| IBIS file stm32u5f9_5g9_lqfp144_dsi_smps.ibs
[IBIS ver] 4.2
[File name] stm32u5f9_5g9_lqfp144_dsi_smps.ibs
[File Rev] 1.0
[Date]  29-10-2024
[Source] Data Created at STMicroelectronics
[Notes]  File originated from ELDO simulations.
[Disclaimer]  This information is for modeling purpose only and is
   not guaranteed. The information is subject to change without
   notice.
[Copyright] Copyright 2024 STMicroelectronics Inc.
|   Component stm32u5f9_5g9_lqfp144_dsi_smps
[Component] stm32u5f9_5g9_lqfp144_dsi_smps
[Manufacturer] STMicroelectronics
[Package]
| variable   typ   min   max
R_pkg  0  NA  NA
L_pkg  0  NA  NA
C_pkg  0  NA  NA
[Pin]   signal_name   model_name
1 PE2 io8_100m_hslv_ft
2 PE3 io8_100m_hslv_tamp_ft
3 PE4 io8_100m_hslv_tamp_ft
4 PE5 io8_100m_hslv_tamp_ft
5 PE6 io8_100m_hslv_tamp_ft
6 VBAT power
7 PC13 io8_100m_ft_v33
8 PC14-OSC32_IN  io8_100m_ft
9 PC15-OSC32_OUT io8_100m_ft
10 PF0 io8_100m_hslv_ft
11 PF1 io8_100m_hslv_ft
12 PF2 io8_100m_hslv_ft
13 VDDDSI nc
14 VDD11DSI nc
15 DSI_D0P nc
16 DSI_D0N nc
17 VSSDSI nc
18 DSI_CKP nc
19 DSI_CKN nc
20 VDD11DSI nc
21 DSI_D1P nc
22 DSI_D1N nc
23 VSSDSI nc
24 VSS gnd
25 VDD power
26 PH0-OSC_IN io8_100m_ft
27 PH1-OSC_OUT io8_100m_ft
28 NRST nc
29 PC0 io8_100m_hslv_ft
30 PC1 io8_166m_hslv_i2c_ft
31 PC2 io8_100m_hslv_ft
32 PC3 io8_100m_hslv_ft
33 VSSA nc
34 VREFP nc
35 VDDA nc
36 PA0 io8_100m_hslv_tamp_ft
37 PA1 io8_100m_hslv_tamp_ft
38 PA2 io8_100m_hslv_ft
39 PA3 io8_166m_hslv_ft
40 VSS gnd
41 VDD power
42 PA4 io8_100m_hslv_ft
43 PA5 io8_100m_ft
44 PA6 io8_100m_hslv_ft
45 PA7 io8_100m_hslv_ft
46 PB0 io8_100m_hslv_ft
47 PB1 io8_100m_hslv_ft
48 PB2 io8_100m_hslv_tamp_ft
49 PG0 io8_100m_hslv_ft
50 PG1 io8_100m_hslv_ft
51 PE7 io8_100m_hslv_ft
52 PE8 io8_100m_hslv_ft
53 PE9 io8_166m_hslv_ft
54 VSS gnd
55 VDD power
56 PE10 io8_166m_hslv_ft
57 PE11 io8_100m_hslv_ft
58 PE12 io8_100m_hslv_ft
59 PE13 io8_100m_hslv_ft
60 PE14 io8_100m_hslv_ft
61 PE15 io8_100m_hslv_ft
62 PB10 io8_166m_hslv_i2c_ft
63 PB11 io8_100m_hslv_ft
64 VLXSMPS nc
65 VDDSMPS nc
66 VSSSMPS nc
67 VDD11 nc
68 VSS gnd
69 VDD power
70 PB13 io8_100m_i2c_ft
71 PB14 io8_100m_hslv_ft
72 PB15 nc
73 PD8 io8_100m_hslv_ft
74 PD9 io8_100m_hslv_ft
75 PD10 io8_100m_hslv_ft
76 PD11 io8_100m_hslv_ft
77 PD12 io8_100m_hslv_ft
78 PD13 io8_100m_hslv_ft
79 PD14 io8_100m_hslv_ft
80 PD15 io8_100m_hslv_ft
81 PH9 io8_spi_ft
82 VSS gnd
83 VDD power
84 PH10 io8_spi_ft
85 PH11 io8_spi_ft
86 PH12 io8_spi_ft
87 PH13 io8_spi_ft
88 VSS gnd
89 VDD power
90 PH14 io8_spi_ft
91 PH15 io8_spi_ft
92 PI0 io8_spi_ft
93 PI1 io8_spi_ft
94 VSS gnd
95 VDD power
96 PI2 io8_spi_ft
97 PI3 io8_spi_ft
98 PC6 io8_100m_hslv_ft
99 PC7 io8_100m_hslv_ft
100 PC8 io8_100m_hslv_ft
101 PC9 io8_100m_hslv_ft
102 PA8 io8_166m_hslv_ft
103 PA9 io8_100m_usb_vbus_ft
104 PA10 io8_100m_usb_id
105 PA11 io8_100m_ft
106 PA12 io8_100m_ft
107 PA13 io8_100m_ft
108 VDDUSB power
109 VDD power
110 VSS gnd
111 PA14 io8_100m_ft
112 PA15 nc
113 PC10 io8_100m_hslv_ft
114 PC11 io8_100m_hslv_ft
115 PC12 io8_166m_hslv_ft
116 PD0 io8_100m_hslv_ft
117 PD1 io8_100m_hslv_ft
118 PD2 io8_100m_hslv_ft
119 PD3 io8_166m_hslv_ft
120 PD4 io8_100m_hslv_ft
121 PD5 io8_100m_hslv_ft
122 VDD power
123 PD6 io8_166m_hslv_ft
124 PD7 io8_100m_hslv_ft
125 PG9 io8_100m_hslv_ft
126 PG10 io8_100m_hslv_ft
127 PG12 io8_100m_hslv_ft
128 PG13 io8_100m_hslv_ft
129 PG14 io8_100m_hslv_ft
130 VSS gnd
131 VDDIO2 power
132 PG15 io8_100m_hslv_ft
133 PB3 io8_100m_hslv_ft
134 PB4 io8_100m_hslv_ft
135 PB5 io8_166m_hslv_ft
136 PB6 io8_100m_i2c_ft
137 PB7 io8_166m_hslv_i2c_ft
138 PH3-BOOT0 io8_100m_ft
139 PB8 io8_100m_hslv_ft
140 PB9 io8_100m_hslv_ft
141 PE0 io8_100m_hslv_ft
142 VDD11 nc
143 VSS gnd
144 VDD power
[Package Model]   476-lqfp-20x20-144-smps-dsi-220916
[Pin Mapping]   pulldown_ref   pullup_ref   | Comment
19  nc  nc
18  nc  nc
16  nc  nc
15  nc  nc
22  nc  nc
21  nc  nc
28  nc  nc
36  gndio  vddiom
37  gndio  vddiom
104  gndio  vddiom  | Depending on IO usage
| 104  gndio  vddusb  | Depending on IO usage
105  gndio  vddiom  | Depending on IO usage
| 105  gndio  vddusb  | Depending on IO usage
106  gndio  vddiom  | Depending on IO usage
| 106  gndio  vddusb  | Depending on IO usage
107  gndio  vddiom  | Depending on IO usage
| 107  gndio  vddusb  | Depending on IO usage
111  gndio  vddiom
112  nc  nc
38  gndio  vddiom
39  gndio  vddiom
42  gndio  vddiom
43  gndio  vddiom
44  gndio  vddiom
45  gndio  vddiom
102  gndio  vddiom
103  gndio  vddiom  | Depending on IO usage
| 103  gndio  vddusb  | Depending on IO usage
46  gndio  vddiom
47  gndio  vddiom
62  gndio  vddiom
63  gndio  vddiom
70  gndio  vddiom
71  gndio  vddiom
72  nc  nc
48  gndio  vddiom
133  gndio  vddiom
134  gndio  vddiom
135  gndio  vddiom
136  gndio  vddiom
137  gndio  vddiom
139  gndio  vddiom
140  gndio  vddiom
29  gndio  vddiom
30  gndio  vddiom
113  gndio  vddiom
114  gndio  vddiom
115  gndio  vddiom
7  gndio  vddiom  | Depending on IO usage
| 7  gndio  vsw  | Depending on IO usage
8  gndio  vddiom  | Depending on IO usage
| 8  gndio  vsw  | Depending on IO usage
9  gndio  vddiom  | Depending on IO usage
| 9  gndio  vsw  | Depending on IO usage
31  gndio  vddiom
32  gndio  vddiom
98  gndio  vddiom
99  gndio  vddiom
100  gndio  vddiom
101  gndio  vddiom
116  gndio  vddiom
117  gndio  vddiom
75  gndio  vddiom
76  gndio  vddiom
77  gndio  vddiom
78  gndio  vddiom
79  gndio  vddiom
80  gndio  vddiom
118  gndio  vddiom
119  gndio  vddiom
120  gndio  vddiom
121  gndio  vddiom
123  gndio  vddiom
124  gndio  vddiom
73  gndio  vddiom
74  gndio  vddiom
141  gndio  vddiom
56  gndio  vddiom
57  gndio  vddiom
58  gndio  vddiom
59  gndio  vddiom
60  gndio  vddiom
61  gndio  vddiom
1  gndio  vddiom
2  gndio  vddiom
3  gndio  vddiom
4  gndio  vddiom
5  gndio  vddiom
51  gndio  vddiom
52  gndio  vddiom
53  gndio  vddiom
10  gndio  vddiom
11  gndio  vddiom
12  gndio  vddiom
49  gndio  vddiom
50  gndio  vddiom
126  gndio  vddiom  | Depending on IO usage
| 126  gndio  vddio2  | Depending on IO usage
127  gndio  vddiom  | Depending on IO usage
| 127  gndio  vddio2  | Depending on IO usage
128  gndio  vddiom  | Depending on IO usage
| 128  gndio  vddio2  | Depending on IO usage
129  gndio  vddiom  | Depending on IO usage
| 129  gndio  vddio2  | Depending on IO usage
132  gndio  vddiom  | Depending on IO usage
| 132  gndio  vddio2  | Depending on IO usage
125  gndio  vddiom  | Depending on IO usage
| 125  gndio  vddio2  | Depending on IO usage
26  gndio  vddiom
27  gndio  vddiom
84  gndio  vddiom
85  gndio  vddiom  | Depending on IO usage
| 85  gndio  vddhspi  | Depending on IO usage
86  gndio  vddiom  | Depending on IO usage
| 86  gndio  vddhspi  | Depending on IO usage
87  gndio  vddiom  | Depending on IO usage
| 87  gndio  vddhspi  | Depending on IO usage
90  gndio  vddiom  | Depending on IO usage
| 90  gndio  vddhspi  | Depending on IO usage
91  gndio  vddiom  | Depending on IO usage
| 91  gndio  vddhspi  | Depending on IO usage
138  gndio  vddiom
81  gndio  vddiom  | Depending on IO usage
| 81  gndio  vddhspi  | Depending on IO usage
92  gndio  vddiom  | Depending on IO usage
| 92  gndio  vddhspi  | Depending on IO usage
93  gndio  vddiom  | Depending on IO usage
| 93  gndio  vddhspi  | Depending on IO usage
96  gndio  vddiom  | Depending on IO usage
| 96  gndio  vddhspi  | Depending on IO usage
97  gndio  vddiom  | Depending on IO usage
| 97  gndio  vddhspi  | Depending on IO usage
67  nc  nc
142  nc  nc
6  nc  vsw
83  nc  vddhspi
89  nc  vddhspi
95  nc  vddhspi
13  nc  nc
109  nc  vddiom
14  nc  nc
20  nc  nc
122  nc  vddiom
144  nc  vddiom
25  nc  vddiom
108  nc  vddusb
41  nc  vddiom
55  nc  vddiom
69  nc  vddiom
35  nc  nc
131  nc  vddio2
65  nc  nc
64  nc  nc
34  nc  nc
24  gndio  nc
40  gndio  nc
54  gndio  nc
68  gndio  nc
110  gndio  nc
143  gndio  nc
17  nc  nc
23  nc  nc
130  gndio  nc
82  gndio  nc
88  gndio  nc
94  gndio  nc
33  nc  nc
66  nc  nc
[Model Selector] io8_100m_ft
io8_100m_ft_hs_1v2  "IO8_FT 100MHz high speed @ 1.2V"
io8_100m_ft_fs_1v2  "IO8_FT 100MHz fast speed @ 1.2V"
io8_100m_ft_fs_pd_1v2  "IO8_FT 100MHz fast speed @ 1.2V pulldown"
io8_100m_ft_ms_1v2  "IO8_FT 100MHz med speed @ 1.2V"
io8_100m_ft_ms_pd_1v2  "IO8_FT 100MHz med speed @ 1.2V pulldown"
io8_100m_ft_ls_1v2  "IO8_FT 100MHz low speed @ 1.2V"
io8_100m_ft_ls_pd_1v2  "IO8_FT 100MHz low speed @ 1.2V pulldown"
io8_100m_ft_hs_1v8  "IO8_FT 100MHz high speed @ 1.8V"
io8_100m_ft_hs_pd_1v8  "IO8_FT 100MHz high speed @ 1.8V pulldown"
io8_100m_ft_fs_1v8  "IO8_FT 100MHz fast speed @ 1.8V"
io8_100m_ft_fs_pd_1v8  "IO8_FT 100MHz fast speed @ 1.8V pulldown"
io8_100m_ft_ms_1v8  "IO8_FT 100MHz med speed @ 1.8V"
io8_100m_ft_ms_pd_1v8  "IO8_FT 100MHz med speed @ 1.8V pulldown"
io8_100m_ft_ls_1v8  "IO8_FT 100MHz low speed @ 1.8V"
io8_100m_ft_ls_pd_1v8  "IO8_FT 100MHz low speed @ 1.8V pulldown"
io8_100m_ft_hs_3v3  "IO8_FT 100MHz high speed @ 3.3V"
io8_100m_ft_hs_pd_3v3  "IO8_FT 100MHz high speed @ 3.3V pulldown"
io8_100m_ft_fs_3v3  "IO8_FT 100MHz fast speed @ 3.3V"
io8_100m_ft_fs_pd_3v3  "IO8_FT 100MHz fast speed @ 3.3V pulldown"
io8_100m_ft_ms_3v3  "IO8_FT 100MHz med speed @ 3.3V"
io8_100m_ft_ms_pd_3v3  "IO8_FT 100MHz med speed @ 3.3V pulldown"
io8_100m_ft_ls_3v3  "IO8_FT 100MHz low speed @ 3.3V"
io8_100m_ft_ls_pd_3v3  "IO8_FT 100MHz low speed @ 3.3V pulldown"
[Model Selector] io8_100m_hslv_ft
io8_100m_ft_hs_1v2  "IO8_FT 100MHz high speed @ 1.2V"
io8_100m_ft_hs_pu_1v2  "IO8_FT 100MHz high speed @ 1.2V pullup"
io8_100m_ft_hs_pd_1v2  "IO8_FT 100MHz high speed @ 1.2V pulldown"
io8_100m_ft_fs_1v2  "IO8_FT 100MHz fast speed @ 1.2V"
io8_100m_ft_fs_pu_1v2  "IO8_FT 100MHz fast speed @ 1.2V pullup"
io8_100m_ft_fs_pd_1v2  "IO8_FT 100MHz fast speed @ 1.2V pulldown"
io8_100m_ft_ms_1v2  "IO8_FT 100MHz med speed @ 1.2V"
io8_100m_ft_ms_pu_1v2  "IO8_FT 100MHz med speed @ 1.2V pullup"
io8_100m_ft_ms_pd_1v2  "IO8_FT 100MHz med speed @ 1.2V pulldown"
io8_100m_ft_ls_1v2  "IO8_FT 100MHz low speed @ 1.2V"
io8_100m_ft_ls_pu_1v2  "IO8_FT 100MHz low speed @ 1.2V pullup"
io8_100m_ft_ls_pd_1v2  "IO8_FT 100MHz low speed @ 1.2V pulldown"
io8_100m_ft_hs_1v8  "IO8_FT 100MHz high speed @ 1.8V"
io8_100m_ft_hs_pu_1v8  "IO8_FT 100MHz high speed @ 1.8V pullup"
io8_100m_ft_hs_pd_1v8  "IO8_FT 100MHz high speed @ 1.8V pulldown"
io8_100m_ft_fs_1v8  "IO8_FT 100MHz fast speed @ 1.8V"
io8_100m_ft_fs_pu_1v8  "IO8_FT 100MHz fast speed @ 1.8V pullup"
io8_100m_ft_fs_pd_1v8  "IO8_FT 100MHz fast speed @ 1.8V pulldown"
io8_100m_ft_ms_1v8  "IO8_FT 100MHz med speed @ 1.8V"
io8_100m_ft_ms_pu_1v8  "IO8_FT 100MHz med speed @ 1.8V pullup"
io8_100m_ft_ms_pd_1v8  "IO8_FT 100MHz med speed @ 1.8V pulldown"
io8_100m_ft_ls_1v8  "IO8_FT 100MHz low speed @ 1.8V"
io8_100m_ft_ls_pu_1v8  "IO8_FT 100MHz low speed @ 1.8V pullup"
io8_100m_ft_ls_pd_1v8  "IO8_FT 100MHz low speed @ 1.8V pulldown"
io8_100m_ft_hs_3v3  "IO8_FT 100MHz high speed @ 3.3V"
io8_100m_ft_hs_pu_3v3  "IO8_FT 100MHz high speed @ 3.3V pullup"
io8_100m_ft_hs_pd_3v3  "IO8_FT 100MHz high speed @ 3.3V pulldown"
io8_100m_ft_fs_3v3  "IO8_FT 100MHz fast speed @ 3.3V"
io8_100m_ft_fs_pu_3v3  "IO8_FT 100MHz fast speed @ 3.3V pullup"
io8_100m_ft_fs_pd_3v3  "IO8_FT 100MHz fast speed @ 3.3V pulldown"
io8_100m_ft_ms_3v3  "IO8_FT 100MHz med speed @ 3.3V"
io8_100m_ft_ms_pu_3v3  "IO8_FT 100MHz med speed @ 3.3V pullup"
io8_100m_ft_ms_pd_3v3  "IO8_FT 100MHz med speed @ 3.3V pulldown"
io8_100m_ft_ls_3v3  "IO8_FT 100MHz low speed @ 3.3V"
io8_100m_ft_ls_pu_3v3  "IO8_FT 100MHz low speed @ 3.3V pullup"
io8_100m_ft_ls_pd_3v3  "IO8_FT 100MHz low speed @ 3.3V pulldown"
io8_100m_hslv_ft_hs_1v2  "IO8_FT 100MHz HSLV high speed @ 1.2V"
io8_100m_hslv_ft_hs_pu_1v2  "IO8_FT 100MHz HSLV high speed @ 1.2V pullup"
io8_100m_hslv_ft_hs_pd_1v2  "IO8_FT 100MHz HSLV high speed @ 1.2V pulldown"
io8_100m_hslv_ft_fs_1v2  "IO8_FT 100MHz HSLV fast speed @ 1.2V"
io8_100m_hslv_ft_fs_pu_1v2  "IO8_FT 100MHz HSLV fast speed @ 1.2V pullup"
io8_100m_hslv_ft_fs_pd_1v2  "IO8_FT 100MHz HSLV fast speed @ 1.2V pulldown"
io8_100m_hslv_ft_ms_1v2  "IO8_FT 100MHz HSLV med speed @ 1.2V"
io8_100m_hslv_ft_ms_pu_1v2  "IO8_FT 100MHz HSLV med speed @ 1.2V pullup"
io8_100m_hslv_ft_ms_pd_1v2  "IO8_FT 100MHz HSLV med speed @ 1.2V pulldown"
io8_100m_hslv_ft_ls_1v2  "IO8_FT 100MHz HSLV low speed @ 1.2V"
io8_100m_hslv_ft_ls_pu_1v2  "IO8_FT 100MHz HSLV low speed @ 1.2V pullup"
io8_100m_hslv_ft_ls_pd_1v2  "IO8_FT 100MHz HSLV low speed @ 1.2V pulldown"
io8_100m_hslv_ft_hs_1v8  "IO8_FT 100MHz HSLV high speed @ 1.8V"
io8_100m_hslv_ft_hs_pu_1v8  "IO8_FT 100MHz HSLV high speed @ 1.8V pullup"
io8_100m_hslv_ft_hs_pd_1v8  "IO8_FT 100MHz HSLV high speed @ 1.8V pulldown"
io8_100m_hslv_ft_fs_1v8  "IO8_FT 100MHz HSLV fast speed @ 1.8V"
io8_100m_hslv_ft_fs_pu_1v8  "IO8_FT 100MHz HSLV fast speed @ 1.8V pullup"
io8_100m_hslv_ft_fs_pd_1v8  "IO8_FT 100MHz HSLV fast speed @ 1.8V pulldown"
io8_100m_hslv_ft_ms_1v8  "IO8_FT 100MHz HSLV med speed @ 1.8V"
io8_100m_hslv_ft_ms_pu_1v8  "IO8_FT 100MHz HSLV med speed @ 1.8V pullup"
io8_100m_hslv_ft_ms_pd_1v8  "IO8_FT 100MHz HSLV med speed @ 1.8V pulldown"
io8_100m_hslv_ft_ls_1v8  "IO8_FT 100MHz HSLV low speed @ 1.8V"
io8_100m_hslv_ft_ls_pu_1v8  "IO8_FT 100MHz HSLV low speed @ 1.8V pullup"
io8_100m_hslv_ft_ls_pd_1v8  "IO8_FT 100MHz HSLV low speed @ 1.8V pulldown"
io8_100m_hslv_ft_hs_2v5  "IO8_FT 100MHz HSLV high speed @ 2.5V"
io8_100m_hslv_ft_hs_pu_2v5  "IO8_FT 100MHz HSLV high speed @ 2.5V pullup"
io8_100m_hslv_ft_hs_pd_2v5  "IO8_FT 100MHz HSLV high speed @ 2.5V pulldown"
io8_100m_hslv_ft_fs_2v5  "IO8_FT 100MHz HSLV fast speed @ 2.5V"
io8_100m_hslv_ft_fs_pu_2v5  "IO8_FT 100MHz HSLV fast speed @ 2.5V pullup"
io8_100m_hslv_ft_fs_pd_2v5  "IO8_FT 100MHz HSLV fast speed @ 2.5V pulldown"
io8_100m_hslv_ft_ms_2v5  "IO8_FT 100MHz HSLV med speed @ 2.5V"
io8_100m_hslv_ft_ms_pu_2v5  "IO8_FT 100MHz HSLV med speed @ 2.5V pullup"
io8_100m_hslv_ft_ms_pd_2v5  "IO8_FT 100MHz HSLV med speed @ 2.5V pulldown"
io8_100m_hslv_ft_ls_2v5  "IO8_FT 100MHz HSLV low speed @ 2.5V"
io8_100m_hslv_ft_ls_pu_2v5  "IO8_FT 100MHz HSLV low speed @ 2.5V pullup"
io8_100m_hslv_ft_ls_pd_2v5  "IO8_FT 100MHz HSLV low speed @ 2.5V pulldown"
[Model Selector] io8_100m_hslv_tamp_ft
io8_100m_ft_hs_1v2  "IO8_FT 100MHz high speed @ 1.2V"
io8_100m_ft_hs_pu_1v2  "IO8_FT 100MHz high speed @ 1.2V pullup"
io8_100m_ft_hs_pd_1v2  "IO8_FT 100MHz high speed @ 1.2V pulldown"
io8_100m_ft_fs_1v2  "IO8_FT 100MHz fast speed @ 1.2V"
io8_100m_ft_fs_pu_1v2  "IO8_FT 100MHz fast speed @ 1.2V pullup"
io8_100m_ft_fs_pd_1v2  "IO8_FT 100MHz fast speed @ 1.2V pulldown"
io8_100m_ft_ms_1v2  "IO8_FT 100MHz med speed @ 1.2V"
io8_100m_ft_ms_pu_1v2  "IO8_FT 100MHz med speed @ 1.2V pullup"
io8_100m_ft_ms_pd_1v2  "IO8_FT 100MHz med speed @ 1.2V pulldown"
io8_100m_ft_ls_1v2  "IO8_FT 100MHz low speed @ 1.2V"
io8_100m_ft_ls_pu_1v2  "IO8_FT 100MHz low speed @ 1.2V pullup"
io8_100m_ft_ls_pd_1v2  "IO8_FT 100MHz low speed @ 1.2V pulldown"
io8_100m_ft_hs_1v8  "IO8_FT 100MHz high speed @ 1.8V"
io8_100m_ft_hs_pu_1v8  "IO8_FT 100MHz high speed @ 1.8V pullup"
io8_100m_ft_hs_pd_1v8  "IO8_FT 100MHz high speed @ 1.8V pulldown"
io8_100m_ft_fs_1v8  "IO8_FT 100MHz fast speed @ 1.8V"
io8_100m_ft_fs_pu_1v8  "IO8_FT 100MHz fast speed @ 1.8V pullup"
io8_100m_ft_fs_pd_1v8  "IO8_FT 100MHz fast speed @ 1.8V pulldown"
io8_100m_ft_ms_1v8  "IO8_FT 100MHz med speed @ 1.8V"
io8_100m_ft_ms_pu_1v8  "IO8_FT 100MHz med speed @ 1.8V pullup"
io8_100m_ft_ms_pd_1v8  "IO8_FT 100MHz med speed @ 1.8V pulldown"
io8_100m_ft_ls_1v8  "IO8_FT 100MHz low speed @ 1.8V"
io8_100m_ft_ls_pu_1v8  "IO8_FT 100MHz low speed @ 1.8V pullup"
io8_100m_ft_ls_pd_1v8  "IO8_FT 100MHz low speed @ 1.8V pulldown"
io8_100m_ft_hs_3v3  "IO8_FT 100MHz high speed @ 3.3V"
io8_100m_ft_hs_pu_3v3  "IO8_FT 100MHz high speed @ 3.3V pullup"
io8_100m_ft_hs_pd_3v3  "IO8_FT 100MHz high speed @ 3.3V pulldown"
io8_100m_ft_fs_3v3  "IO8_FT 100MHz fast speed @ 3.3V"
io8_100m_ft_fs_pu_3v3  "IO8_FT 100MHz fast speed @ 3.3V pullup"
io8_100m_ft_fs_pd_3v3  "IO8_FT 100MHz fast speed @ 3.3V pulldown"
io8_100m_ft_ms_3v3  "IO8_FT 100MHz med speed @ 3.3V"
io8_100m_ft_ms_pu_3v3  "IO8_FT 100MHz med speed @ 3.3V pullup"
io8_100m_ft_ms_pd_3v3  "IO8_FT 100MHz med speed @ 3.3V pulldown"
io8_100m_ft_ls_3v3  "IO8_FT 100MHz low speed @ 3.3V"
io8_100m_ft_ls_pu_3v3  "IO8_FT 100MHz low speed @ 3.3V pullup"
io8_100m_ft_ls_pd_3v3  "IO8_FT 100MHz low speed @ 3.3V pulldown"
io8_100m_hslv_ft_hs_1v2  "IO8_FT 100MHz HSLV high speed @ 1.2V"
io8_100m_hslv_ft_hs_pu_1v2  "IO8_FT 100MHz HSLV high speed @ 1.2V pullup"
io8_100m_hslv_ft_hs_pd_1v2  "IO8_FT 100MHz HSLV high speed @ 1.2V pulldown"
io8_100m_hslv_ft_fs_1v2  "IO8_FT 100MHz HSLV fast speed @ 1.2V"
io8_100m_hslv_ft_fs_pu_1v2  "IO8_FT 100MHz HSLV fast speed @ 1.2V pullup"
io8_100m_hslv_ft_fs_pd_1v2  "IO8_FT 100MHz HSLV fast speed @ 1.2V pulldown"
io8_100m_hslv_ft_ms_1v2  "IO8_FT 100MHz HSLV med speed @ 1.2V"
io8_100m_hslv_ft_ms_pu_1v2  "IO8_FT 100MHz HSLV med speed @ 1.2V pullup"
io8_100m_hslv_ft_ms_pd_1v2  "IO8_FT 100MHz HSLV med speed @ 1.2V pulldown"
io8_100m_hslv_ft_ls_1v2  "IO8_FT 100MHz HSLV low speed @ 1.2V"
io8_100m_hslv_ft_ls_pu_1v2  "IO8_FT 100MHz HSLV low speed @ 1.2V pullup"
io8_100m_hslv_ft_ls_pd_1v2  "IO8_FT 100MHz HSLV low speed @ 1.2V pulldown"
io8_100m_hslv_ft_hs_1v8  "IO8_FT 100MHz HSLV high speed @ 1.8V"
io8_100m_hslv_ft_hs_pu_1v8  "IO8_FT 100MHz HSLV high speed @ 1.8V pullup"
io8_100m_hslv_ft_hs_pd_1v8  "IO8_FT 100MHz HSLV high speed @ 1.8V pulldown"
io8_100m_hslv_ft_fs_1v8  "IO8_FT 100MHz HSLV fast speed @ 1.8V"
io8_100m_hslv_ft_fs_pu_1v8  "IO8_FT 100MHz HSLV fast speed @ 1.8V pullup"
io8_100m_hslv_ft_fs_pd_1v8  "IO8_FT 100MHz HSLV fast speed @ 1.8V pulldown"
io8_100m_hslv_ft_ms_1v8  "IO8_FT 100MHz HSLV med speed @ 1.8V"
io8_100m_hslv_ft_ms_pu_1v8  "IO8_FT 100MHz HSLV med speed @ 1.8V pullup"
io8_100m_hslv_ft_ms_pd_1v8  "IO8_FT 100MHz HSLV med speed @ 1.8V pulldown"
io8_100m_hslv_ft_ls_1v8  "IO8_FT 100MHz HSLV low speed @ 1.8V"
io8_100m_hslv_ft_ls_pu_1v8  "IO8_FT 100MHz HSLV low speed @ 1.8V pullup"
io8_100m_hslv_ft_ls_pd_1v8  "IO8_FT 100MHz HSLV low speed @ 1.8V pulldown"
io8_100m_hslv_ft_hs_2v5  "IO8_FT 100MHz HSLV high speed @ 2.5V"
io8_100m_hslv_ft_hs_pu_2v5  "IO8_FT 100MHz HSLV high speed @ 2.5V pullup"
io8_100m_hslv_ft_hs_pd_2v5  "IO8_FT 100MHz HSLV high speed @ 2.5V pulldown"
io8_100m_hslv_ft_fs_2v5  "IO8_FT 100MHz HSLV fast speed @ 2.5V"
io8_100m_hslv_ft_fs_pu_2v5  "IO8_FT 100MHz HSLV fast speed @ 2.5V pullup"
io8_100m_hslv_ft_fs_pd_2v5  "IO8_FT 100MHz HSLV fast speed @ 2.5V pulldown"
io8_100m_hslv_ft_ms_2v5  "IO8_FT 100MHz HSLV med speed @ 2.5V"
io8_100m_hslv_ft_ms_pu_2v5  "IO8_FT 100MHz HSLV med speed @ 2.5V pullup"
io8_100m_hslv_ft_ms_pd_2v5  "IO8_FT 100MHz HSLV med speed @ 2.5V pulldown"
io8_100m_hslv_ft_ls_2v5  "IO8_FT 100MHz HSLV low speed @ 2.5V"
io8_100m_hslv_ft_ls_pu_2v5  "IO8_FT 100MHz HSLV low speed @ 2.5V pullup"
io8_100m_hslv_ft_ls_pd_2v5  "IO8_FT 100MHz HSLV low speed @ 2.5V pulldown"
io8_ft_v33_hs_1v2  "IO8_FT_V33 high speed @ 1.2V"
io8_ft_v33_hs_pu_1v2  "IO8_FT_V33 high speed @ 1.2V pullup"
io8_ft_v33_hs_pd_1v2  "IO8_FT_V33 high speed @ 1.2V pulldown"
io8_ft_v33_fs_1v2  "IO8_FT_V33 fast speed @ 1.2V"
io8_ft_v33_fs_pu_1v2  "IO8_FT_V33 fast speed @ 1.2V pullup"
io8_ft_v33_fs_pd_1v2  "IO8_FT_V33 fast speed @ 1.2V pulldown"
io8_ft_v33_ms_1v2  "IO8_FT_V33 med speed @ 1.2V"
io8_ft_v33_ms_pu_1v2  "IO8_FT_V33 med speed @ 1.2V pullup"
io8_ft_v33_ms_pd_1v2  "IO8_FT_V33 med speed @ 1.2V pulldown"
io8_ft_v33_ls_1v2  "IO8_FT_V33 low speed @ 1.2V"
io8_ft_v33_ls_pu_1v2  "IO8_FT_V33 low speed @ 1.2V pullup"
io8_ft_v33_ls_pd_1v2  "IO8_FT_V33 low speed @ 1.2V pulldown"
io8_ft_v33_hs_1v8  "IO8_FT_V33 high speed @ 1.8V"
io8_ft_v33_hs_pu_1v8  "IO8_FT_V33 high speed @ 1.8V pullup"
io8_ft_v33_hs_pd_1v8  "IO8_FT_V33 high speed @ 1.8V pulldown"
io8_ft_v33_fs_1v8  "IO8_FT_V33 fast speed @ 1.8V"
io8_ft_v33_fs_pu_1v8  "IO8_FT_V33 fast speed @ 1.8V pullup"
io8_ft_v33_fs_pd_1v8  "IO8_FT_V33 fast speed @ 1.8V pulldown"
io8_ft_v33_ms_1v8  "IO8_FT_V33 med speed @ 1.8V"
io8_ft_v33_ms_pu_1v8  "IO8_FT_V33 med speed @ 1.8V pullup"
io8_ft_v33_ms_pd_1v8  "IO8_FT_V33 med speed @ 1.8V pulldown"
io8_ft_v33_ls_1v8  "IO8_FT_V33 low speed @ 1.8V"
io8_ft_v33_ls_pu_1v8  "IO8_FT_V33 low speed @ 1.8V pullup"
io8_ft_v33_ls_pd_1v8  "IO8_FT_V33 low speed @ 1.8V pulldown"
io8_ft_v33_hs_3v3  "IO8_FT_V33 high speed @ 3.3V"
io8_ft_v33_hs_pu_3v3  "IO8_FT_V33 high speed @ 3.3V pullup"
io8_ft_v33_hs_pd_3v3  "IO8_FT_V33 high speed @ 3.3V pulldown"
io8_ft_v33_fs_3v3  "IO8_FT_V33 fast speed @ 3.3V"
io8_ft_v33_fs_pu_3v3  "IO8_FT_V33 fast speed @ 3.3V pullup"
io8_ft_v33_fs_pd_3v3  "IO8_FT_V33 fast speed @ 3.3V pulldown"
io8_ft_v33_ms_3v3  "IO8_FT_V33 med speed @ 3.3V"
io8_ft_v33_ms_pu_3v3  "IO8_FT_V33 med speed @ 3.3V pullup"
io8_ft_v33_ms_pd_3v3  "IO8_FT_V33 med speed @ 3.3V pulldown"
io8_ft_v33_ls_3v3  "IO8_FT_V33 low speed @ 3.3V"
io8_ft_v33_ls_pu_3v3  "IO8_FT_V33 low speed @ 3.3V pullup"
io8_ft_v33_ls_pd_3v3  "IO8_FT_V33 low speed @ 3.3V pulldown"
[Model Selector] io8_100m_i2c_ft
io8_100m_ft_hs_1v2  "IO8_FT 100MHz high speed @ 1.2V"
io8_100m_ft_hs_pu_1v2  "IO8_FT 100MHz high speed @ 1.2V pullup"
io8_100m_ft_hs_pd_1v2  "IO8_FT 100MHz high speed @ 1.2V pulldown"
io8_100m_ft_fs_1v2  "IO8_FT 100MHz fast speed @ 1.2V"
io8_100m_ft_fs_pu_1v2  "IO8_FT 100MHz fast speed @ 1.2V pullup"
io8_100m_ft_fs_pd_1v2  "IO8_FT 100MHz fast speed @ 1.2V pulldown"
io8_100m_ft_ms_1v2  "IO8_FT 100MHz med speed @ 1.2V"
io8_100m_ft_ms_pu_1v2  "IO8_FT 100MHz med speed @ 1.2V pullup"
io8_100m_ft_ms_pd_1v2  "IO8_FT 100MHz med speed @ 1.2V pulldown"
io8_100m_ft_ls_1v2  "IO8_FT 100MHz low speed @ 1.2V"
io8_100m_ft_ls_pu_1v2  "IO8_FT 100MHz low speed @ 1.2V pullup"
io8_100m_ft_ls_pd_1v2  "IO8_FT 100MHz low speed @ 1.2V pulldown"
io8_100m_ft_hs_1v8  "IO8_FT 100MHz high speed @ 1.8V"
io8_100m_ft_hs_pu_1v8  "IO8_FT 100MHz high speed @ 1.8V pullup"
io8_100m_ft_hs_pd_1v8  "IO8_FT 100MHz high speed @ 1.8V pulldown"
io8_100m_ft_fs_1v8  "IO8_FT 100MHz fast speed @ 1.8V"
io8_100m_ft_fs_pu_1v8  "IO8_FT 100MHz fast speed @ 1.8V pullup"
io8_100m_ft_fs_pd_1v8  "IO8_FT 100MHz fast speed @ 1.8V pulldown"
io8_100m_ft_ms_1v8  "IO8_FT 100MHz med speed @ 1.8V"
io8_100m_ft_ms_pu_1v8  "IO8_FT 100MHz med speed @ 1.8V pullup"
io8_100m_ft_ms_pd_1v8  "IO8_FT 100MHz med speed @ 1.8V pulldown"
io8_100m_ft_ls_1v8  "IO8_FT 100MHz low speed @ 1.8V"
io8_100m_ft_ls_pu_1v8  "IO8_FT 100MHz low speed @ 1.8V pullup"
io8_100m_ft_ls_pd_1v8  "IO8_FT 100MHz low speed @ 1.8V pulldown"
io8_100m_ft_hs_3v3  "IO8_FT 100MHz high speed @ 3.3V"
io8_100m_ft_hs_pu_3v3  "IO8_FT 100MHz high speed @ 3.3V pullup"
io8_100m_ft_hs_pd_3v3  "IO8_FT 100MHz high speed @ 3.3V pulldown"
io8_100m_ft_fs_3v3  "IO8_FT 100MHz fast speed @ 3.3V"
io8_100m_ft_fs_pu_3v3  "IO8_FT 100MHz fast speed @ 3.3V pullup"
io8_100m_ft_fs_pd_3v3  "IO8_FT 100MHz fast speed @ 3.3V pulldown"
io8_100m_ft_ms_3v3  "IO8_FT 100MHz med speed @ 3.3V"
io8_100m_ft_ms_pu_3v3  "IO8_FT 100MHz med speed @ 3.3V pullup"
io8_100m_ft_ms_pd_3v3  "IO8_FT 100MHz med speed @ 3.3V pulldown"
io8_100m_ft_ls_3v3  "IO8_FT 100MHz low speed @ 3.3V"
io8_100m_ft_ls_pu_3v3  "IO8_FT 100MHz low speed @ 3.3V pullup"
io8_100m_ft_ls_pd_3v3  "IO8_FT 100MHz low speed @ 3.3V pulldown"
io8_100m_i2c_ft_1v2  "IO8_FT 100MHz I2C @ 1.2V"
io8_100m_i2c_ft_pu_1v2  "IO8_FT 100MHz I2C @ 1.2V pullup"
io8_100m_i2c_ft_pd_1v2  "IO8_FT 100MHz I2C @ 1.2V pulldown"
io8_100m_i2c_ft_1v8  "IO8_FT 100MHz I2C @ 1.8V"
io8_100m_i2c_ft_pu_1v8  "IO8_FT 100MHz I2C @ 1.8V pullup"
io8_100m_i2c_ft_pd_1v8  "IO8_FT 100MHz I2C @ 1,8V pulldown"
io8_100m_i2c_ft_3v3  "IO8_FT 100MHz I2C @ 3.3V"
io8_100m_i2c_ft_pu_3v3  "IO8_FT 100MHz I2C HSLV @ 3.3V pullup"
io8_100m_i2c_ft_pd_3v3  "IO8_FT 100MHz I2C @ 3.3V pulldown"
[Model Selector] io8_100m_usb_id
io8_100m_ft_hs_1v2  "IO8_FT 100MHz high speed @ 1.2V"
io8_100m_ft_hs_pu_1v2  "IO8_FT 100MHz high speed @ 1.2V pullup"
io8_100m_ft_hs_pd_1v2  "IO8_FT 100MHz high speed @ 1.2V pulldown"
io8_100m_ft_fs_1v2  "IO8_FT 100MHz fast speed @ 1.2V"
io8_100m_ft_fs_pu_1v2  "IO8_FT 100MHz fast speed @ 1.2V pullup"
io8_100m_ft_fs_pd_1v2  "IO8_FT 100MHz fast speed @ 1.2V pulldown"
io8_100m_ft_ms_1v2  "IO8_FT 100MHz med speed @ 1.2V"
io8_100m_ft_ms_pu_1v2  "IO8_FT 100MHz med speed @ 1.2V pullup"
io8_100m_ft_ms_pd_1v2  "IO8_FT 100MHz med speed @ 1.2V pulldown"
io8_100m_ft_ls_1v2  "IO8_FT 100MHz low speed @ 1.2V"
io8_100m_ft_ls_pu_1v2  "IO8_FT 100MHz low speed @ 1.2V pullup"
io8_100m_ft_ls_pd_1v2  "IO8_FT 100MHz low speed @ 1.2V pulldown"
io8_100m_ft_hs_1v8  "IO8_FT 100MHz high speed @ 1.8V"
io8_100m_ft_hs_pu_1v8  "IO8_FT 100MHz high speed @ 1.8V pullup"
io8_100m_ft_hs_pd_1v8  "IO8_FT 100MHz high speed @ 1.8V pulldown"
io8_100m_ft_fs_1v8  "IO8_FT 100MHz fast speed @ 1.8V"
io8_100m_ft_fs_pu_1v8  "IO8_FT 100MHz fast speed @ 1.8V pullup"
io8_100m_ft_fs_pd_1v8  "IO8_FT 100MHz fast speed @ 1.8V pulldown"
io8_100m_ft_ms_1v8  "IO8_FT 100MHz med speed @ 1.8V"
io8_100m_ft_ms_pu_1v8  "IO8_FT 100MHz med speed @ 1.8V pullup"
io8_100m_ft_ms_pd_1v8  "IO8_FT 100MHz med speed @ 1.8V pulldown"
io8_100m_ft_ls_1v8  "IO8_FT 100MHz low speed @ 1.8V"
io8_100m_ft_ls_pu_1v8  "IO8_FT 100MHz low speed @ 1.8V pullup"
io8_100m_ft_ls_pd_1v8  "IO8_FT 100MHz low speed @ 1.8V pulldown"
io8_100m_ft_hs_3v3  "IO8_FT 100MHz high speed @ 3.3V"
io8_100m_ft_hs_pu_3v3  "IO8_FT 100MHz high speed @ 3.3V pullup"
io8_100m_ft_hs_pd_3v3  "IO8_FT 100MHz high speed @ 3.3V pulldown"
io8_100m_ft_fs_3v3  "IO8_FT 100MHz fast speed @ 3.3V"
io8_100m_ft_fs_pu_3v3  "IO8_FT 100MHz fast speed @ 3.3V pullup"
io8_100m_ft_fs_pd_3v3  "IO8_FT 100MHz fast speed @ 3.3V pulldown"
io8_100m_ft_ms_3v3  "IO8_FT 100MHz med speed @ 3.3V"
io8_100m_ft_ms_pu_3v3  "IO8_FT 100MHz med speed @ 3.3V pullup"
io8_100m_ft_ms_pd_3v3  "IO8_FT 100MHz med speed @ 3.3V pulldown"
io8_100m_ft_ls_3v3  "IO8_FT 100MHz low speed @ 3.3V"
io8_100m_ft_ls_pu_3v3  "IO8_FT 100MHz low speed @ 3.3V pullup"
io8_100m_ft_ls_pd_3v3  "IO8_FT 100MHz low speed @ 3.3V pulldown"
io8usb_id_nopu  "IOUSB ID @ 3.3V"
io8usb_id_pu  "IOUSB ID @ 3.3V pullup"
[Model Selector] io8_100m_usb_vbus_ft
io8_100m_ft_hs_1v2  "IO8_FT 100MHz high speed @ 1.2V"
io8_100m_ft_hs_pu_1v2  "IO8_FT 100MHz high speed @ 1.2V pullup"
io8_100m_ft_hs_pd_1v2  "IO8_FT 100MHz high speed @ 1.2V pulldown"
io8_100m_ft_fs_1v2  "IO8_FT 100MHz fast speed @ 1.2V"
io8_100m_ft_fs_pu_1v2  "IO8_FT 100MHz fast speed @ 1.2V pullup"
io8_100m_ft_fs_pd_1v2  "IO8_FT 100MHz fast speed @ 1.2V pulldown"
io8_100m_ft_ms_1v2  "IO8_FT 100MHz med speed @ 1.2V"
io8_100m_ft_ms_pu_1v2  "IO8_FT 100MHz med speed @ 1.2V pullup"
io8_100m_ft_ms_pd_1v2  "IO8_FT 100MHz med speed @ 1.2V pulldown"
io8_100m_ft_ls_1v2  "IO8_FT 100MHz low speed @ 1.2V"
io8_100m_ft_ls_pu_1v2  "IO8_FT 100MHz low speed @ 1.2V pullup"
io8_100m_ft_ls_pd_1v2  "IO8_FT 100MHz low speed @ 1.2V pulldown"
io8_100m_ft_hs_1v8  "IO8_FT 100MHz high speed @ 1.8V"
io8_100m_ft_hs_pu_1v8  "IO8_FT 100MHz high speed @ 1.8V pullup"
io8_100m_ft_hs_pd_1v8  "IO8_FT 100MHz high speed @ 1.8V pulldown"
io8_100m_ft_fs_1v8  "IO8_FT 100MHz fast speed @ 1.8V"
io8_100m_ft_fs_pu_1v8  "IO8_FT 100MHz fast speed @ 1.8V pullup"
io8_100m_ft_fs_pd_1v8  "IO8_FT 100MHz fast speed @ 1.8V pulldown"
io8_100m_ft_ms_1v8  "IO8_FT 100MHz med speed @ 1.8V"
io8_100m_ft_ms_pu_1v8  "IO8_FT 100MHz med speed @ 1.8V pullup"
io8_100m_ft_ms_pd_1v8  "IO8_FT 100MHz med speed @ 1.8V pulldown"
io8_100m_ft_ls_1v8  "IO8_FT 100MHz low speed @ 1.8V"
io8_100m_ft_ls_pu_1v8  "IO8_FT 100MHz low speed @ 1.8V pullup"
io8_100m_ft_ls_pd_1v8  "IO8_FT 100MHz low speed @ 1.8V pulldown"
io8_100m_ft_hs_3v3  "IO8_FT 100MHz high speed @ 3.3V"
io8_100m_ft_hs_pu_3v3  "IO8_FT 100MHz high speed @ 3.3V pullup"
io8_100m_ft_hs_pd_3v3  "IO8_FT 100MHz high speed @ 3.3V pulldown"
io8_100m_ft_fs_3v3  "IO8_FT 100MHz fast speed @ 3.3V"
io8_100m_ft_fs_pu_3v3  "IO8_FT 100MHz fast speed @ 3.3V pullup"
io8_100m_ft_fs_pd_3v3  "IO8_FT 100MHz fast speed @ 3.3V pulldown"
io8_100m_ft_ms_3v3  "IO8_FT 100MHz med speed @ 3.3V"
io8_100m_ft_ms_pu_3v3  "IO8_FT 100MHz med speed @ 3.3V pullup"
io8_100m_ft_ms_pd_3v3  "IO8_FT 100MHz med speed @ 3.3V pulldown"
io8_100m_ft_ls_3v3  "IO8_FT 100MHz low speed @ 3.3V"
io8_100m_ft_ls_pu_3v3  "IO8_FT 100MHz low speed @ 3.3V pullup"
io8_100m_ft_ls_pd_3v3  "IO8_FT 100MHz low speed @ 3.3V pulldown"
io8usb_adp "IOUSB ADP @ 3.3V"
io8usb_vbus "IOUSB VBUS @ 3.3V"
[Model Selector] io8_166m_hslv_ft
io8_166m_ft_hs_1v2  "IO8_FT 166MHz high speed @ 1.2V"
io8_166m_ft_hs_pu_1v2  "IO8_FT 166MHz high speed @ 1.2V pullup"
io8_166m_ft_hs_pd_1v2  "IO8_FT 166MHz high speed @ 1.2V pulldown"
io8_166m_ft_fs_1v2  "IO8_FT 166MHz fast speed @ 1.2V"
io8_166m_ft_fs_pu_1v2  "IO8_FT 166MHz fast speed @ 1.2V pullup"
io8_166m_ft_fs_pd_1v2  "IO8_FT 166MHz fast speed @ 1.2V pulldown"
io8_166m_ft_ms_1v2  "IO8_FT 166MHz med speed @ 1.2V"
io8_166m_ft_ms_pu_1v2  "IO8_FT 166MHz med speed @ 1.2V pullup"
io8_166m_ft_ms_pd_1v2  "IO8_FT 166MHz med speed @ 1.2V pulldown"
io8_166m_ft_ls_1v2  "IO8_FT 166MHz low speed @ 1.2V"
io8_166m_ft_ls_pu_1v2  "IO8_FT 166MHz low speed @ 1.2V pullup"
io8_166m_ft_ls_pd_1v2  "IO8_FT 166MHz low speed @ 1.2V pulldown"
io8_166m_ft_hs_1v8  "IO8_FT 166MHz high speed @ 1.8V"
io8_166m_ft_hs_pu_1v8  "IO8_FT 166MHz high speed @ 1.8V pullup"
io8_166m_ft_hs_pd_1v8  "IO8_FT 166MHz high speed @ 1.8V pulldown"
io8_166m_ft_fs_1v8  "IO8_FT 166MHz fast speed @ 1.8V"
io8_166m_ft_fs_pu_1v8  "IO8_FT 166MHz fast speed @ 1.8V pullup"
io8_166m_ft_fs_pd_1v8  "IO8_FT 166MHz fast speed @ 1.8V pulldown"
io8_166m_ft_ms_1v8  "IO8_FT 166MHz med speed @ 1.8V"
io8_166m_ft_ms_pu_1v8  "IO8_FT 166MHz med speed @ 1.8V pullup"
io8_166m_ft_ms_pd_1v8  "IO8_FT 166MHz med speed @ 1.8V pulldown"
io8_166m_ft_ls_1v8  "IO8_FT 166MHz low speed @ 1.8V"
io8_166m_ft_ls_pu_1v8  "IO8_FT 166MHz low speed @ 1.8V pullup"
io8_166m_ft_ls_pd_1v8  "IO8_FT 166MHz low speed @ 1.8V pulldown"
io8_166m_ft_hs_3v3  "IO8_FT 166MHz high speed @ 3.3V"
io8_166m_ft_hs_pu_3v3  "IO8_FT 166MHz high speed @ 3.3V pullup"
io8_166m_ft_hs_pd_3v3  "IO8_FT 166MHz high speed @ 3.3V pulldown"
io8_166m_ft_fs_3v3  "IO8_FT 166MHz fast speed @ 3.3V"
io8_166m_ft_fs_pu_3v3  "IO8_FT 166MHz fast speed @ 3.3V pullup"
io8_166m_ft_fs_pd_3v3  "IO8_FT 166MHz fast speed @ 3.3V pulldown"
io8_166m_ft_ms_3v3  "IO8_FT 166MHz med speed @ 3.3V"
io8_166m_ft_ms_pu_3v3  "IO8_FT 166MHz med speed @ 3.3V pullup"
io8_166m_ft_ms_pd_3v3  "IO8_FT 166MHz med speed @ 3.3V pulldown"
io8_166m_ft_ls_3v3  "IO8_FT 166MHz low speed @ 3.3V"
io8_166m_ft_ls_pu_3v3  "IO8_FT 166MHz low speed @ 3.3V pullup"
io8_166m_ft_ls_pd_3v3  "IO8_FT 166MHz low speed @ 3.3V pulldown"
io8_166m_hslv_ft_hs_1v2  "IO8_FT 166MHz HSLV high speed @ 1.2V"
io8_166m_hslv_ft_hs_pu_1v2  "IO8_FT 166MHz HSLV high speed @ 1.2V pullup"
io8_166m_hslv_ft_hs_pd_1v2  "IO8_FT 166MHz HSLV high speed @ 1.2V pulldown"
io8_166m_hslv_ft_fs_1v2  "IO8_FT 166MHz HSLV fast speed @ 1.2V"
io8_166m_hslv_ft_fs_pu_1v2  "IO8_FT 166MHz HSLV fast speed @ 1.2V pullup"
io8_166m_hslv_ft_fs_pd_1v2  "IO8_FT 166MHz HSLV fast speed @ 1.2V pulldown"
io8_166m_hslv_ft_ms_1v2  "IO8_FT 166MHz HSLV med speed @ 1.2V"
io8_166m_hslv_ft_ms_pu_1v2  "IO8_FT 166MHz HSLV med speed @ 1.2V pullup"
io8_166m_hslv_ft_ms_pd_1v2  "IO8_FT 166MHz HSLV med speed @ 1.2V pulldown"
io8_166m_hslv_ft_ls_1v2  "IO8_FT 166MHz HSLV low speed @ 1.2V"
io8_166m_hslv_ft_ls_pu_1v2  "IO8_FT 166MHz HSLV low speed @ 1.2V pullup"
io8_166m_hslv_ft_ls_pd_1v2  "IO8_FT 166MHz HSLV low speed @ 1.2V pulldown"
io8_166m_hslv_ft_hs_1v8  "IO8_FT 166MHz HSLV high speed @ 1.8V"
io8_166m_hslv_ft_hs_pu_1v8  "IO8_FT 166MHz HSLV high speed @ 1.8V pullup"
io8_166m_hslv_ft_hs_pd_1v8  "IO8_FT 166MHz HSLV high speed @ 1.8V pulldown"
io8_166m_hslv_ft_fs_1v8  "IO8_FT 166MHz HSLV fast speed @ 1.8V"
io8_166m_hslv_ft_fs_pu_1v8  "IO8_FT 166MHz HSLV fast speed @ 1.8V pullup"
io8_166m_hslv_ft_fs_pd_1v8  "IO8_FT 166MHz HSLV fast speed @ 1.8V pulldown"
io8_166m_hslv_ft_ms_1v8  "IO8_FT 166MHz HSLV med speed @ 1.8V"
io8_166m_hslv_ft_ms_pu_1v8  "IO8_FT 166MHz HSLV med speed @ 1.8V pullup"
io8_166m_hslv_ft_ms_pd_1v8  "IO8_FT 166MHz HSLV med speed @ 1.8V pulldown"
io8_166m_hslv_ft_ls_1v8  "IO8_FT 166MHz HSLV low speed @ 1.8V"
io8_166m_hslv_ft_ls_pu_1v8  "IO8_FT 166MHz HSLV low speed @ 1.8V pullup"
io8_166m_hslv_ft_ls_pd_1v8  "IO8_FT 166MHz HSLV low speed @ 1.8V pulldown"
io8_166m_hslv_ft_hs_2v5  "IO8_FT 166MHz HSLV high speed @ 2.5V"
io8_166m_hslv_ft_hs_pu_2v5  "IO8_FT 166MHz HSLV high speed @ 2.5V pullup"
io8_166m_hslv_ft_hs_pd_2v5  "IO8_FT 166MHz HSLV high speed @ 2.5V pulldown"
io8_166m_hslv_ft_fs_2v5  "IO8_FT 166MHz HSLV fast speed @ 2.5V"
io8_166m_hslv_ft_fs_pu_2v5  "IO8_FT 166MHz HSLV fast speed @ 2.5V pullup"
io8_166m_hslv_ft_fs_pd_2v5  "IO8_FT 166MHz HSLV fast speed @ 2.5V pulldown"
io8_166m_hslv_ft_ms_2v5  "IO8_FT 166MHz HSLV med speed @ 2.5V"
io8_166m_hslv_ft_ms_pu_2v5  "IO8_FT 166MHz HSLV med speed @ 2.5V pullup"
io8_166m_hslv_ft_ms_pd_2v5  "IO8_FT 166MHz HSLV med speed @ 2.5V pulldown"
io8_166m_hslv_ft_ls_2v5  "IO8_FT 166MHz HSLV low speed @ 2.5V"
io8_166m_hslv_ft_ls_pu_2v5  "IO8_FT 166MHz HSLV low speed @ 2.5V pullup"
io8_166m_hslv_ft_ls_pd_2v5  "IO8_FT 166MHz HSLV low speed @ 2.5V pulldown"
[Model Selector] io8_166m_hslv_i2c_ft
io8_166m_ft_hs_1v2  "IO8_FT 166MHz high speed @ 1.2V"
io8_166m_ft_hs_pu_1v2  "IO8_FT 166MHz high speed @ 1.2V pullup"
io8_166m_ft_hs_pd_1v2  "IO8_FT 166MHz high speed @ 1.2V pulldown"
io8_166m_ft_fs_1v2  "IO8_FT 166MHz fast speed @ 1.2V"
io8_166m_ft_fs_pu_1v2  "IO8_FT 166MHz fast speed @ 1.2V pullup"
io8_166m_ft_fs_pd_1v2  "IO8_FT 166MHz fast speed @ 1.2V pulldown"
io8_166m_ft_ms_1v2  "IO8_FT 166MHz med speed @ 1.2V"
io8_166m_ft_ms_pu_1v2  "IO8_FT 166MHz med speed @ 1.2V pullup"
io8_166m_ft_ms_pd_1v2  "IO8_FT 166MHz med speed @ 1.2V pulldown"
io8_166m_ft_ls_1v2  "IO8_FT 166MHz low speed @ 1.2V"
io8_166m_ft_ls_pu_1v2  "IO8_FT 166MHz low speed @ 1.2V pullup"
io8_166m_ft_ls_pd_1v2  "IO8_FT 166MHz low speed @ 1.2V pulldown"
io8_166m_ft_hs_1v8  "IO8_FT 166MHz high speed @ 1.8V"
io8_166m_ft_hs_pu_1v8  "IO8_FT 166MHz high speed @ 1.8V pullup"
io8_166m_ft_hs_pd_1v8  "IO8_FT 166MHz high speed @ 1.8V pulldown"
io8_166m_ft_fs_1v8  "IO8_FT 166MHz fast speed @ 1.8V"
io8_166m_ft_fs_pu_1v8  "IO8_FT 166MHz fast speed @ 1.8V pullup"
io8_166m_ft_fs_pd_1v8  "IO8_FT 166MHz fast speed @ 1.8V pulldown"
io8_166m_ft_ms_1v8  "IO8_FT 166MHz med speed @ 1.8V"
io8_166m_ft_ms_pu_1v8  "IO8_FT 166MHz med speed @ 1.8V pullup"
io8_166m_ft_ms_pd_1v8  "IO8_FT 166MHz med speed @ 1.8V pulldown"
io8_166m_ft_ls_1v8  "IO8_FT 166MHz low speed @ 1.8V"
io8_166m_ft_ls_pu_1v8  "IO8_FT 166MHz low speed @ 1.8V pullup"
io8_166m_ft_ls_pd_1v8  "IO8_FT 166MHz low speed @ 1.8V pulldown"
io8_166m_ft_hs_3v3  "IO8_FT 166MHz high speed @ 3.3V"
io8_166m_ft_hs_pu_3v3  "IO8_FT 166MHz high speed @ 3.3V pullup"
io8_166m_ft_hs_pd_3v3  "IO8_FT 166MHz high speed @ 3.3V pulldown"
io8_166m_ft_fs_3v3  "IO8_FT 166MHz fast speed @ 3.3V"
io8_166m_ft_fs_pu_3v3  "IO8_FT 166MHz fast speed @ 3.3V pullup"
io8_166m_ft_fs_pd_3v3  "IO8_FT 166MHz fast speed @ 3.3V pulldown"
io8_166m_ft_ms_3v3  "IO8_FT 166MHz med speed @ 3.3V"
io8_166m_ft_ms_pu_3v3  "IO8_FT 166MHz med speed @ 3.3V pullup"
io8_166m_ft_ms_pd_3v3  "IO8_FT 166MHz med speed @ 3.3V pulldown"
io8_166m_ft_ls_3v3  "IO8_FT 166MHz low speed @ 3.3V"
io8_166m_ft_ls_pu_3v3  "IO8_FT 166MHz low speed @ 3.3V pullup"
io8_166m_ft_ls_pd_3v3  "IO8_FT 166MHz low speed @ 3.3V pulldown"
io8_166m_hslv_ft_hs_1v2  "IO8_FT 166MHz HSLV high speed @ 1.2V"
io8_166m_hslv_ft_hs_pu_1v2  "IO8_FT 166MHz HSLV high speed @ 1.2V pullup"
io8_166m_hslv_ft_hs_pd_1v2  "IO8_FT 166MHz HSLV high speed @ 1.2V pulldown"
io8_166m_hslv_ft_fs_1v2  "IO8_FT 166MHz HSLV fast speed @ 1.2V"
io8_166m_hslv_ft_fs_pu_1v2  "IO8_FT 166MHz HSLV fast speed @ 1.2V pullup"
io8_166m_hslv_ft_fs_pd_1v2  "IO8_FT 166MHz HSLV fast speed @ 1.2V pulldown"
io8_166m_hslv_ft_ms_1v2  "IO8_FT 166MHz HSLV med speed @ 1.2V"
io8_166m_hslv_ft_ms_pu_1v2  "IO8_FT 166MHz HSLV med speed @ 1.2V pullup"
io8_166m_hslv_ft_ms_pd_1v2  "IO8_FT 166MHz HSLV med speed @ 1.2V pulldown"
io8_166m_hslv_ft_ls_1v2  "IO8_FT 166MHz HSLV low speed @ 1.2V"
io8_166m_hslv_ft_ls_pu_1v2  "IO8_FT 166MHz HSLV low speed @ 1.2V pullup"
io8_166m_hslv_ft_ls_pd_1v2  "IO8_FT 166MHz HSLV low speed @ 1.2V pulldown"
io8_166m_hslv_ft_hs_1v8  "IO8_FT 166MHz HSLV high speed @ 1.8V"
io8_166m_hslv_ft_hs_pu_1v8  "IO8_FT 166MHz HSLV high speed @ 1.8V pullup"
io8_166m_hslv_ft_hs_pd_1v8  "IO8_FT 166MHz HSLV high speed @ 1.8V pulldown"
io8_166m_hslv_ft_fs_1v8  "IO8_FT 166MHz HSLV fast speed @ 1.8V"
io8_166m_hslv_ft_fs_pu_1v8  "IO8_FT 166MHz HSLV fast speed @ 1.8V pullup"
io8_166m_hslv_ft_fs_pd_1v8  "IO8_FT 166MHz HSLV fast speed @ 1.8V pulldown"
io8_166m_hslv_ft_ms_1v8  "IO8_FT 166MHz HSLV med speed @ 1.8V"
io8_166m_hslv_ft_ms_pu_1v8  "IO8_FT 166MHz HSLV med speed @ 1.8V pullup"
io8_166m_hslv_ft_ms_pd_1v8  "IO8_FT 166MHz HSLV med speed @ 1.8V pulldown"
io8_166m_hslv_ft_ls_1v8  "IO8_FT 166MHz HSLV low speed @ 1.8V"
io8_166m_hslv_ft_ls_pu_1v8  "IO8_FT 166MHz HSLV low speed @ 1.8V pullup"
io8_166m_hslv_ft_ls_pd_1v8  "IO8_FT 166MHz HSLV low speed @ 1.8V pulldown"
io8_166m_hslv_ft_hs_2v5  "IO8_FT 166MHz HSLV high speed @ 2.5V"
io8_166m_hslv_ft_hs_pu_2v5  "IO8_FT 166MHz HSLV high speed @ 2.5V pullup"
io8_166m_hslv_ft_hs_pd_2v5  "IO8_FT 166MHz HSLV high speed @ 2.5V pulldown"
io8_166m_hslv_ft_fs_2v5  "IO8_FT 166MHz HSLV fast speed @ 2.5V"
io8_166m_hslv_ft_fs_pu_2v5  "IO8_FT 166MHz HSLV fast speed @ 2.5V pullup"
io8_166m_hslv_ft_fs_pd_2v5  "IO8_FT 166MHz HSLV fast speed @ 2.5V pulldown"
io8_166m_hslv_ft_ms_2v5  "IO8_FT 166MHz HSLV med speed @ 2.5V"
io8_166m_hslv_ft_ms_pu_2v5  "IO8_FT 166MHz HSLV med speed @ 2.5V pullup"
io8_166m_hslv_ft_ms_pd_2v5  "IO8_FT 166MHz HSLV med speed @ 2.5V pulldown"
io8_166m_hslv_ft_ls_2v5  "IO8_FT 166MHz HSLV low speed @ 2.5V"
io8_166m_hslv_ft_ls_pu_2v5  "IO8_FT 166MHz HSLV low speed @ 2.5V pullup"
io8_166m_hslv_ft_ls_pd_2v5  "IO8_FT 166MHz HSLV low speed @ 2.5V pulldown"
io8_166m_i2c_ft_1v2  "IO8_FT 166MHz I2C @ 1.2V"
io8_166m_i2c_ft_pu_1v2  "IO8_FT 166MHz I2C @ 1.2V pullup"
io8_166m_i2c_ft_pd_1v2  "IO8_FT 166MHz I2C @ 1.2V pulldown"
io8_166m_i2c_ft_1v8  "IO8_FT 166MHz I2C @ 1.8V"
io8_166m_i2c_ft_pu_1v8  "IO8_FT 166MHz I2C @ 1.8V pullup"
io8_166m_i2c_ft_pd_1v8  "IO8_FT 166MHz I2C @ 1,8V pulldown"
io8_166m_i2c_ft_3v3  "IO8_FT 166MHz I2C @ 3.3V"
io8_166m_i2c_ft_pu_3v3  "IO8_FT 166MHz I2C HSLV @ 3.3V pullup"
io8_166m_i2c_ft_pd_3v3  "IO8_FT 166MHz I2C @ 3.3V pulldown"
[Model Selector] io8_100m_ft_v33
io8_ft_v33_hs_1v2  "IO8_FT_V33 high speed @ 1.2V"
io8_ft_v33_hs_pu_1v2  "IO8_FT_V33 high speed @ 1.2V pullup"
io8_ft_v33_hs_pd_1v2  "IO8_FT_V33 high speed @ 1.2V pulldown"
io8_ft_v33_fs_1v2  "IO8_FT_V33 fast speed @ 1.2V"
io8_ft_v33_fs_pu_1v2  "IO8_FT_V33 fast speed @ 1.2V pullup"
io8_ft_v33_fs_pd_1v2  "IO8_FT_V33 fast speed @ 1.2V pulldown"
io8_ft_v33_ms_1v2  "IO8_FT_V33 med speed @ 1.2V"
io8_ft_v33_ms_pu_1v2  "IO8_FT_V33 med speed @ 1.2V pullup"
io8_ft_v33_ms_pd_1v2  "IO8_FT_V33 med speed @ 1.2V pulldown"
io8_ft_v33_ls_1v2  "IO8_FT_V33 low speed @ 1.2V"
io8_ft_v33_ls_pu_1v2  "IO8_FT_V33 low speed @ 1.2V pullup"
io8_ft_v33_ls_pd_1v2  "IO8_FT_V33 low speed @ 1.2V pulldown"
io8_ft_v33_hs_1v8  "IO8_FT_V33 high speed @ 1.8V"
io8_ft_v33_hs_pu_1v8  "IO8_FT_V33 high speed @ 1.8V pullup"
io8_ft_v33_hs_pd_1v8  "IO8_FT_V33 high speed @ 1.8V pulldown"
io8_ft_v33_fs_1v8  "IO8_FT_V33 fast speed @ 1.8V"
io8_ft_v33_fs_pu_1v8  "IO8_FT_V33 fast speed @ 1.8V pullup"
io8_ft_v33_fs_pd_1v8  "IO8_FT_V33 fast speed @ 1.8V pulldown"
io8_ft_v33_ms_1v8  "IO8_FT_V33 med speed @ 1.8V"
io8_ft_v33_ms_pu_1v8  "IO8_FT_V33 med speed @ 1.8V pullup"
io8_ft_v33_ms_pd_1v8  "IO8_FT_V33 med speed @ 1.8V pulldown"
io8_ft_v33_ls_1v8  "IO8_FT_V33 low speed @ 1.8V"
io8_ft_v33_ls_pu_1v8  "IO8_FT_V33 low speed @ 1.8V pullup"
io8_ft_v33_ls_pd_1v8  "IO8_FT_V33 low speed @ 1.8V pulldown"
io8_ft_v33_hs_3v3  "IO8_FT_V33 high speed @ 3.3V"
io8_ft_v33_hs_pu_3v3  "IO8_FT_V33 high speed @ 3.3V pullup"
io8_ft_v33_hs_pd_3v3  "IO8_FT_V33 high speed @ 3.3V pulldown"
io8_ft_v33_fs_3v3  "IO8_FT_V33 fast speed @ 3.3V"
io8_ft_v33_fs_pu_3v3  "IO8_FT_V33 fast speed @ 3.3V pullup"
io8_ft_v33_fs_pd_3v3  "IO8_FT_V33 fast speed @ 3.3V pulldown"
io8_ft_v33_ms_3v3  "IO8_FT_V33 med speed @ 3.3V"
io8_ft_v33_ms_pu_3v3  "IO8_FT_V33 med speed @ 3.3V pullup"
io8_ft_v33_ms_pd_3v3  "IO8_FT_V33 med speed @ 3.3V pulldown"
io8_ft_v33_ls_3v3  "IO8_FT_V33 low speed @ 3.3V"
io8_ft_v33_ls_pu_3v3  "IO8_FT_V33 low speed @ 3.3V pullup"
io8_ft_v33_ls_pd_3v3  "IO8_FT_V33 low speed @ 3.3V pulldown"
[Model Selector] io8_spi_ft
io8_spi_ft_hs_1v2  "IO8_FT SPI high speed @ 1.2V"
io8_spi_ft_hs_pu_1v2  "IO8_FT SPI high speed @ 1.2V pullup"
io8_spi_ft_hs_pd_1v2  "IO8_FT SPI high speed @ 1.2V pulldown"
io8_spi_ft_fs_1v2  "IO8_FT SPI fast speed @ 1.2V"
io8_spi_ft_fs_pu_1v2  "IO8_FT SPI fast speed @ 1.2V pullup"
io8_spi_ft_fs_pd_1v2  "IO8_FT SPI fast speed @ 1.2V pulldown"
io8_spi_ft_ms_1v2  "IO8_FT SPI med speed @ 1.2V"
io8_spi_ft_ms_pu_1v2  "IO8_FT SPI med speed @ 1.2V pullup"
io8_spi_ft_ms_pd_1v2  "IO8_FT SPI med speed @ 1.2V pulldown"
io8_spi_ft_ls_1v2  "IO8_FT SPI low speed @ 1.2V"
io8_spi_ft_ls_pu_1v2  "IO8_FT SPI low speed @ 1.2V pullup"
io8_spi_ft_ls_pd_1v2  "IO8_FT SPI low speed @ 1.2V pulldown"
io8_spi_ft_hs_1v8  "IO8_FT SPI high speed @ 1.8V"
io8_spi_ft_hs_pu_1v8  "IO8_FT SPI high speed @ 1.8V pullup"
io8_spi_ft_hs_pd_1v8  "IO8_FT SPI high speed @ 1.8V pulldown"
io8_spi_ft_fs_1v8  "IO8_FT SPI fast speed @ 1.8V"
io8_spi_ft_fs_pu_1v8  "IO8_FT SPI fast speed @ 1.8V pullup"
io8_spi_ft_fs_pd_1v8  "IO8_FT SPI fast speed @ 1.8V pulldown"
io8_spi_ft_ms_1v8  "IO8_FT SPI med speed @ 1.8V"
io8_spi_ft_ms_pu_1v8  "IO8_FT SPI med speed @ 1.8V pullup"
io8_spi_ft_ms_pd_1v8  "IO8_FT SPI med speed @ 1.8V pulldown"
io8_spi_ft_ls_1v8  "IO8_FT SPI low speed @ 1.8V"
io8_spi_ft_ls_pu_1v8  "IO8_FT SPI low speed @ 1.8V pullup"
io8_spi_ft_ls_pd_1v8  "IO8_FT SPI low speed @ 1.8V pulldown"
io8_spi_ft_hs_3v3  "IO8_FT SPI high speed @ 3.3V"
io8_spi_ft_hs_pu_3v3  "IO8_FT SPI high speed @ 3.3V pullup"
io8_spi_ft_hs_pd_3v3  "IO8_FT SPI high speed @ 3.3V pulldown"
io8_spi_ft_fs_3v3  "IO8_FT SPI fast speed @ 3.3V"
io8_spi_ft_fs_pu_3v3  "IO8_FT SPI fast speed @ 3.3V pullup"
io8_spi_ft_fs_pd_3v3  "IO8_FT SPI fast speed @ 3.3V pulldown"
io8_spi_ft_ms_3v3  "IO8_FT SPI med speed @ 3.3V"
io8_spi_ft_ms_pu_3v3  "IO8_FT SPI med speed @ 1.8V pullup"
io8_spi_ft_ms_pd_3v3  "IO8_FT SPI med speed @ 3.3V pulldown"
io8_spi_ft_ls_3v3  "IO8_FT SPI low speed @ 3.3V"
io8_spi_ft_ls_pu_3v3  "IO8_FT SPI low speed @ 3.3V pullup"
io8_spi_ft_ls_pd_3v3  "IO8_FT SPI low speed @ 3.3V pulldown"
io8_spi_hslv_ft_hs_1v2  "IO8_FT SPI HSLV high speed @ 1.2V"
io8_spi_hslv_ft_hs_pu_1v2  "IO8_FT SPI HSLV high speed @ 1.2V pullup"
io8_spi_hslv_ft_hs_pd_1v2  "IO8_FT SPI HSLV high speed @ 1.2V pulldown"
io8_spi_hslv_ft_fs_1v2  "IO8_FT SPI HSLV fast speed @ 1.2V"
io8_spi_hslv_ft_fs_pu_1v2  "IO8_FT SPI HSLV fast speed @ 1.2V pullup"
io8_spi_hslv_ft_fs_pd_1v2  "IO8_FT SPI HSLV fast speed @ 1.2V pulldown"
io8_spi_hslv_ft_ms_1v2  "IO8_FT SPI HSLV med speed @ 1.2V"
io8_spi_hslv_ft_ms_pu_1v2  "IO8_FT SPI HSLV med speed @ 1.2V pullup"
io8_spi_hslv_ft_ms_pd_1v2  "IO8_FT SPI HSLV med speed @ 1.2V pulldown"
io8_spi_hslv_ft_ls_1v2  "IO8_FT SPI HSLV low speed @ 1.2V"
io8_spi_hslv_ft_ls_pu_1v2  "IO8_FT SPI HSLV low speed @ 1.2V pullup"
io8_spi_hslv_ft_ls_pd_1v2  "IO8_FT SPI HSLV low speed @ 1.2V pulldown"
io8_spi_hslv_ft_hs_1v8  "IO8_FT SPI HSLV high speed @ 1.8V"
io8_spi_hslv_ft_hs_pu_1v8  "IO8_FT SPI HSLV high speed @ 1.8V pullup"
io8_spi_hslv_ft_hs_pd_1v8  "IO8_FT SPI HSLV high speed @ 1.8V pulldown"
io8_spi_hslv_ft_fs_1v8  "IO8_FT SPI HSLV fast speed @ 1.8V"
io8_spi_hslv_ft_fs_pu_1v8  "IO8_FT SPI HSLV fast speed @ 1.8V pullup"
io8_spi_hslv_ft_fs_pd_1v8  "IO8_FT SPI HSLV fast speed @ 1.8V pulldown"
io8_spi_hslv_ft_ms_1v8  "IO8_FT SPI HSLV med speed @ 1.8V"
io8_spi_hslv_ft_ms_pu_1v8  "IO8_FT SPI HSLV med speed @ 1.8V pullup"
io8_spi_hslv_ft_ms_pd_1v8  "IO8_FT SPI HSLV med speed @ 1.8V pulldown"
io8_spi_hslv_ft_ls_1v8  "IO8_FT SPI HSLV low speed @ 1.8V"
io8_spi_hslv_ft_ls_pu_1v8  "IO8_FT SPI HSLV low speed @ 1.8V pullup"
io8_spi_hslv_ft_ls_pd_1v8  "IO8_FT SPI HSLV low speed @ 1.8V pulldown"
io8_spi_hslv_ft_hs_2v5  "IO8_FT SPI HSLV high speed @ 2.5V"
io8_spi_hslv_ft_hs_pu_2v5  "IO8_FT SPI HSLV high speed @ 2.5V pullup"
io8_spi_hslv_ft_hs_pd_2v5  "IO8_FT SPI HSLV high speed @ 2.5V pulldown"
io8_spi_hslv_ft_fs_2v5  "IO8_FT SPI HSLV fast speed @ 2.5V"
io8_spi_hslv_ft_fs_pu_2v5  "IO8_FT SPI HSLV fast speed @ 2.5V pullup"
io8_spi_hslv_ft_fs_pd_2v5  "IO8_FT SPI HSLV fast speed @ 2.5V pulldown"
io8_spi_hslv_ft_ms_2v5  "IO8_FT SPI HSLV med speed @ 2.5V"
io8_spi_hslv_ft_ms_pu_2v5  "IO8_FT SPI HSLV med speed @ 2.5V pullup"
io8_spi_hslv_ft_ms_pd_2v5  "IO8_FT SPI HSLV med speed @ 2.5V pulldown"
io8_spi_hslv_ft_ls_2v5  "IO8_FT SPI HSLV low speed @ 2.5V"
io8_spi_hslv_ft_ls_pu_2v5  "IO8_FT SPI HSLV low speed @ 2.5V pullup"
io8_spi_hslv_ft_ls_pd_2v5  "IO8_FT SPI HSLV low speed @ 2.5V pulldown"
[Define Package Model]  476-lqfp-20x20-144-smps-dsi-220916
[Manufacturer]  Unknown
[OEM]  Unknown
[Description]  None
[Number Of Pins]  139
[Pin Numbers]
| Pin Num   Terminal Name
19 | DSI_CKN
18 | DSI_CKP
16 | DSI_D0N
15 | DSI_D0P
22 | DSI_D1N
21 | DSI_D1P
28 | NRST
36 | PA0
37 | PA1
38 | PA2
39 | PA3
42 | PA4
43 | PA5
44 | PA6
45 | PA7
102 | PA8
103 | PA9
104 | PA10
105 | PA11
106 | PA12
107 | PA13
111 | PA14
112 | PA15
46 | PB0
47 | PB1
48 | PB2
133 | PB3
134 | PB4
135 | PB5
136 | PB6
137 | PB7
139 | PB8
140 | PB9
62 | PB10
63 | PB11
70 | PB13
71 | PB14
72 | PB15
29 | PC0
30 | PC1
31 | PC2
32 | PC3
98 | PC6
99 | PC7
100 | PC8
101 | PC9
113 | PC10
114 | PC11
115 | PC12
7 | PC13
8 | PC14-OSC32_IN
9 | PC15-OSC32_OUT
116 | PD0
117 | PD1
118 | PD2
119 | PD3
120 | PD4
121 | PD5
123 | PD6
124 | PD7
73 | PD8
74 | PD9
75 | PD10
76 | PD11
77 | PD12
78 | PD13
79 | PD14
80 | PD15
141 | PE0
1 | PE2
2 | PE3
3 | PE4
4 | PE5
5 | PE6
51 | PE7
52 | PE8
53 | PE9
56 | PE10
57 | PE11
58 | PE12
59 | PE13
60 | PE14
61 | PE15
10 | PF0
11 | PF1
12 | PF2
49 | PG0
50 | PG1
125 | PG9
126 | PG10
127 | PG12
128 | PG13
129 | PG14
132 | PG15
26 | PH0-OSC_IN
27 | PH1
138 | PH3-BOOT0
81 | PH9
84 | PH10
85 | PH11
86 | PH12
87 | PH13
90 | PH14
91 | PH15
92 | PI0
93 | PI1
96 | PI2
97 | PI3
67 | VDD11
142 | VDD11
6 | VBAT
83 | VDD
89 | VDD
95 | VDD
13 | VDDDSI
14 | VDD11DSI
20 | VDD11DSI
108 | VDDUSB
25 | VDD
41 | VDD
55 | VDD
69 | VDD
109 | VDD
122 | VDD
144 | VDD
35 | VDDA
131 | VDDIO2
65 | VDDSMPS
64 | VLXSMPS
34 | VREFP
24 | VSS
17 | VSSDSI
23 | VSSDSI
82 | VSS
88 | VSS
94 | VSS
130 | VSS
33 | VSSA
66 | VSSSMPS
|[Merged Pins]  24
|40  |  VSS
|54  |  VSS
|68  |  VSS
|110  |  VSS
|143  |  VSS
[Model Data]
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[End Model Data]
[End Package Model]
| Models and submodels in the file (274): io8_100m_ft_hs_1v2 (I/O), io8_100m_ft_hs_pu_1v2 (I/O), io8_100m_ft_hs_pd_1v2 (I/O), io8_100m_ft_fs_1v2 (I/O), io8_100m_ft_fs_pu_1v2 (I/O), io8_100m_ft_fs_pd_1v2 (I/O), io8_100m_ft_ms_1v2 (I/O), io8_100m_ft_ms_pu_1v2 (I/O), io8_100m_ft_ms_pd_1v2 (I/O), io8_100m_ft_ls_1v2 (I/O), io8_100m_ft_ls_pu_1v2 (I/O), io8_100m_ft_ls_pd_1v2 (I/O), io8_100m_ft_hs_1v8 (I/O), io8_100m_ft_hs_pu_1v8 (I/O), io8_100m_ft_hs_pd_1v8 (I/O), io8_100m_ft_fs_1v8 (I/O), io8_100m_ft_fs_pu_1v8 (I/O), io8_100m_ft_fs_pd_1v8 (I/O), io8_100m_ft_ms_1v8 (I/O), io8_100m_ft_ms_pu_1v8 (I/O), io8_100m_ft_ms_pd_1v8 (I/O), io8_100m_ft_ls_1v8 (I/O), io8_100m_ft_ls_pu_1v8 (I/O), io8_100m_ft_ls_pd_1v8 (I/O), io8_100m_ft_hs_3v3 (I/O), io8_100m_ft_hs_pu_3v3 (I/O), io8_100m_ft_hs_pd_3v3 (I/O), io8_100m_ft_fs_3v3 (I/O), io8_100m_ft_fs_pu_3v3 (I/O), io8_100m_ft_fs_pd_3v3 (I/O), io8_100m_ft_ms_3v3 (I/O), io8_100m_ft_ms_pu_3v3 (I/O), io8_100m_ft_ms_pd_3v3 (I/O), io8_100m_ft_ls_3v3 (I/O), io8_100m_ft_ls_pu_3v3 (I/O), io8_100m_ft_ls_pd_3v3 (I/O), io8_100m_hslv_ft_hs_1v2 (I/O), io8_100m_hslv_ft_hs_pu_1v2 (I/O), io8_100m_hslv_ft_hs_pd_1v2 (I/O), io8_100m_hslv_ft_fs_1v2 (I/O), io8_100m_hslv_ft_fs_pu_1v2 (I/O), io8_100m_hslv_ft_fs_pd_1v2 (I/O), io8_100m_hslv_ft_ms_1v2 (I/O), io8_100m_hslv_ft_ms_pu_1v2 (I/O), io8_100m_hslv_ft_ms_pd_1v2 (I/O), io8_100m_hslv_ft_ls_1v2 (I/O), io8_100m_hslv_ft_ls_pu_1v2 (I/O), io8_100m_hslv_ft_ls_pd_1v2 (I/O), io8_100m_hslv_ft_hs_1v8 (I/O), io8_100m_hslv_ft_hs_pu_1v8 (I/O), io8_100m_hslv_ft_hs_pd_1v8 (I/O), io8_100m_hslv_ft_fs_1v8 (I/O), io8_100m_hslv_ft_fs_pu_1v8 (I/O), io8_100m_hslv_ft_fs_pd_1v8 (I/O), io8_100m_hslv_ft_ms_1v8 (I/O), io8_100m_hslv_ft_ms_pu_1v8 (I/O), io8_100m_hslv_ft_ms_pd_1v8 (I/O), io8_100m_hslv_ft_ls_1v8 (I/O), io8_100m_hslv_ft_ls_pu_1v8 (I/O), io8_100m_hslv_ft_ls_pd_1v8 (I/O), io8_100m_hslv_ft_hs_2v5 (I/O), io8_100m_hslv_ft_hs_pu_2v5 (I/O), io8_100m_hslv_ft_hs_pd_2v5 (I/O), io8_100m_hslv_ft_fs_2v5 (I/O), io8_100m_hslv_ft_fs_pu_2v5 (I/O), io8_100m_hslv_ft_fs_pd_2v5 (I/O), io8_100m_hslv_ft_ms_2v5 (I/O), io8_100m_hslv_ft_ms_pu_2v5 (I/O), io8_100m_hslv_ft_ms_pd_2v5 (I/O), io8_100m_hslv_ft_ls_2v5 (I/O), io8_100m_hslv_ft_ls_pu_2v5 (I/O), io8_100m_hslv_ft_ls_pd_2v5 (I/O), io8_166m_ft_hs_1v2 (I/O), io8_166m_ft_hs_pu_1v2 (I/O), io8_166m_ft_hs_pd_1v2 (I/O), io8_166m_ft_fs_1v2 (I/O), io8_166m_ft_fs_pu_1v2 (I/O), io8_166m_ft_fs_pd_1v2 (I/O), io8_166m_ft_ms_1v2 (I/O), io8_166m_ft_ms_pu_1v2 (I/O)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
